PROGRAM RotaryKnifeApplication
VAR_INPUT
	RegistrationSensor				: BOOL;
END_VAR
VAR
	state							: MotionState_t;
	iTemp							: INT;
	EnableAxes						: BOOL;
	AxesEnabled						: BOOL;
	PowerWebTransport				: MC_Power;
	PowerVirtualWeb					: MC_Power;
	PowerRotaryKnife				: MC_Power;

	CoupleAxes						: BOOL;
	
	GearInVirtualWeb				: MC_GearIn;
	CamInRotaryKnife				: MC_CamIn;

	SetPositionVirtualWeb: MC_SetPosition;
	MoveModuloRotaryKnife: MC_MoveModulo;
	MoveWebTransport: MC_MoveVelocity;
	Halt: MC_Halt;

	TouchProbeRegistration: MC_TouchProbe;
	RegistrationInput : TRIGGER_REF;
	RegistrationError: LREAL;
	ExpectedRegistrationPosition: LREAL;

	MoveSuperImposedVirtualWeb: MC_MoveSuperImposed;
	VirtualWebSyncAngle: LREAL;
	TriggerRegistrationCorrection: R_TRIG;
	TriggerCorrectionFinished : R_TRIG;
	
	lrSlavepos: LREAL;
	
	fbPosTrig:Tc2_Standard.R_TRIG;
END_VAR


(* rotary knife state machine *)

CASE state OF
	MOTIONSTATE_INIT :  //Init
		EnableAxes := FALSE;
		CoupleAxes := FALSE;
		SetPositionVirtualWeb.Execute := FALSE;
		MoveModuloRotaryKnife.Execute := FALSE;
		MoveWebTransport.Execute := FALSE;
		RotaryKnifeCamTable(Execute:=FALSE);
		state := MOTIONSTATE_ADJUSTCAMTABLE ;

	MOTIONSTATE_ADJUSTCAMTABLE :   //CamData
		RotaryKnifeCamTable(Execute:=TRUE , ProductLength:=PRODUCTLENGTH );
		IF RotaryKnifeCamTable.Done THEN
			state := MOTIONSTATE_ENABLE ;
		END_IF

	MOTIONSTATE_ENABLE :        //RegulateOn
		EnableAxes := TRUE;
		IF AxesEnabled THEN
			state := MOTIONSTATE_MOVESLAVE ;
		END_IF

	MOTIONSTATE_MOVESLAVE :   //VirtualMaster to 0 ; Knife Move
		SetPositionVirtualWeb.Execute := TRUE;
		MoveModuloRotaryKnife.Execute := TRUE;
		IF SetPositionVirtualWeb.Done AND MoveModuloRotaryKnife.Done THEN
			state := MOTIONSTATE_COUPLE ;
		END_IF

	MOTIONSTATE_COUPLE :  // Couple  Master Vel With VirtualMaster ;   VirtualMaster Cam With Knife
		CoupleAxes := TRUE;
		IF CamInRotaryKnife.InSync THEN
			state := MOTIONSTATE_START ;
		END_IF

	MOTIONSTATE_START :   // Master Move
		MoveWebTransport.Execute := TRUE;

	MOTIONSTATE_ERROR :
		;
	MOTIONSTATE_RESET :
		;
END_CASE

ActPower();
ActCoupleAxes();
ActMoveSlave();
ActMoveMaster();
ActRegistration();

ACTION ActCoupleAxes:
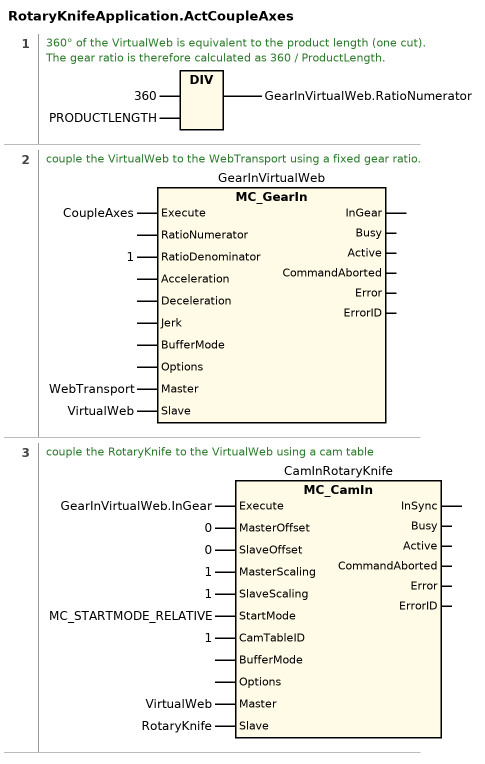
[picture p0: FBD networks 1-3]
// NETWORK 1
// 					360° of the VirtualWeb is equivalent to the product length (one cut).
// The gear ratio is therefore calculated as 360 / ProductLength.
//
GearInVirtualWeb.RatioNumerator := 360 / PRODUCTLENGTH;

// NETWORK 2
// 					couple the VirtualWeb to the WebTransport using a fixed gear ratio.
//
//
GearInVirtualWeb(Execute := CoupleAxes, RatioDenominator := 1, Master := WebTransport, Slave := VirtualWeb); // MC_GearIn

// NETWORK 3
// 					couple the RotaryKnife to the VirtualWeb using a cam table
//
//
CamInRotaryKnife(
    Execute := GearInVirtualWeb.InGear,
    MasterOffset := 0,
    SlaveOffset := 0,
    MasterScaling := 1,
    SlaveScaling := 1,
    StartMode := MC_STARTMODE_RELATIVE,
    CamTableID := 1,
    Master := VirtualWeb,
    Slave := RotaryKnife); // MC_CamIn
END_ACTION

ACTION ActMoveMaster:
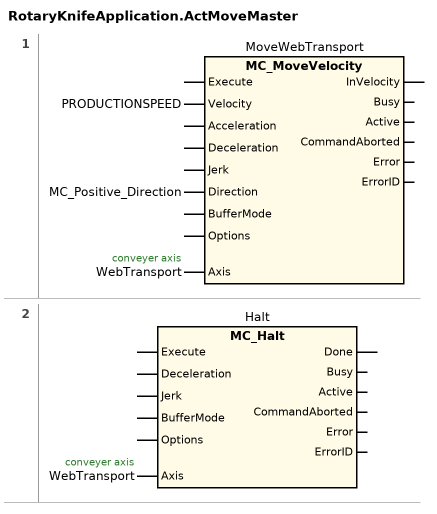
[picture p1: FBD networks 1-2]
// NETWORK 1
//   WebTransport: conveyer axis
MoveWebTransport(Velocity := PRODUCTIONSPEED, Direction := MC_Positive_Direction, Axis := WebTransport); // MC_MoveVelocity

// NETWORK 2
//   WebTransport: conveyer axis
Halt(Axis := WebTransport); // MC_Halt
END_ACTION

ACTION ActMoveSlave:
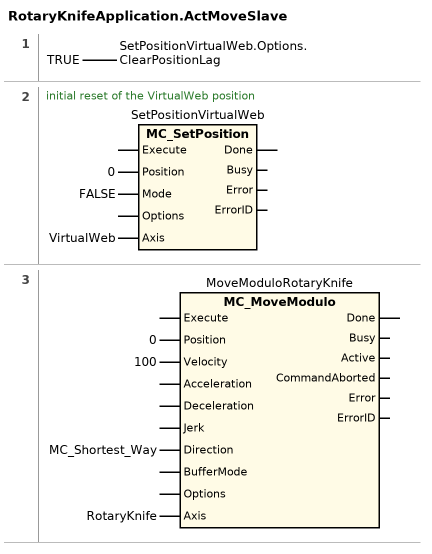
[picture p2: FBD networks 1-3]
// NETWORK 1
SetPositionVirtualWeb.Options.ClearPositionLag := TRUE;

// NETWORK 2
// 					initial reset of the VirtualWeb position
//
//
SetPositionVirtualWeb(Position := 0, Mode := FALSE, Axis := VirtualWeb); // MC_SetPosition

// NETWORK 3
MoveModuloRotaryKnife(Position := 0, Velocity := 100, Direction := MC_Shortest_Way, Axis := RotaryKnife); // MC_MoveModulo
END_ACTION

ACTION ActPower:
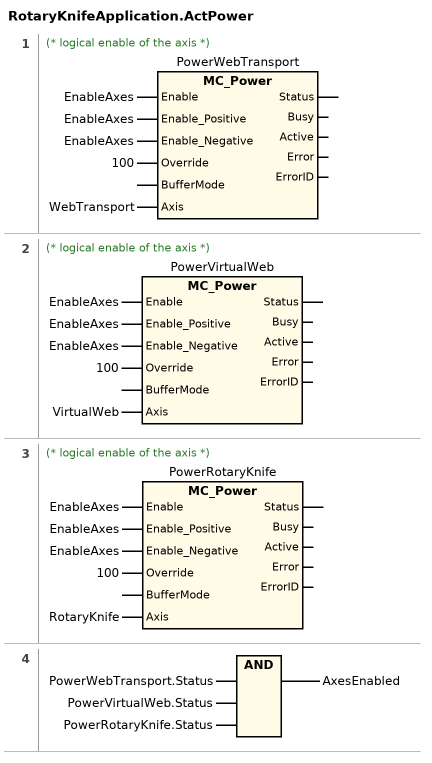
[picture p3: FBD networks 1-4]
// NETWORK 1
// (* logical enable of the axis *)
PowerWebTransport(
    Enable := EnableAxes,
    Enable_Positive := EnableAxes,
    Enable_Negative := EnableAxes,
    Override := 100,
    Axis := WebTransport); // MC_Power

// NETWORK 2
// (* logical enable of the axis *)
PowerVirtualWeb(
    Enable := EnableAxes,
    Enable_Positive := EnableAxes,
    Enable_Negative := EnableAxes,
    Override := 100,
    Axis := VirtualWeb); // MC_Power

// NETWORK 3
// (* logical enable of the axis *)
PowerRotaryKnife(
    Enable := EnableAxes,
    Enable_Positive := EnableAxes,
    Enable_Negative := EnableAxes,
    Override := 100,
    Axis := RotaryKnife); // MC_Power

// NETWORK 4
AxesEnabled := PowerWebTransport.Status AND PowerVirtualWeb.Status AND PowerRotaryKnife.Status;
END_ACTION

ACTION ActRegistration:
(*
 * 	The registration routine detects the registration sensor 
 *	and calculates a position error. The error is corrected by
 *	shifting the VirtualWeb against the WebTransport.
 *)

(* define the touch probe input signal - in this case a simulated signal is used *)
RegistrationInput.Edge := RisingEdge;
RegistrationInput.EncoderID := REGISTRATIONENCODERID;
RegistrationInput.ModuloPositions := TRUE;
RegistrationInput.TouchProbe := PlcEvent; (* use simulated PLC signal, no real probe signal *)

(* feed registration sensor *)
RegistrationInput.PlcEvent := RegistrationSensor; (* simulated PLC signal *)

(* call the registration sensor function block *)
ActRegistrationTouchProbe();

(* calculate a position error after the registration sensor triggered *)
IF 	TouchProbeRegistration.Done	(* new registration value *)
	AND NOT MoveSuperImposedVirtualWeb.Busy (* do not calculate a registration error while correction is busy (wrong measurement) *)
	THEN
	iTemp:=itemp+1;
	ExpectedRegistrationPosition := (PRODUCTLENGTH - REGISTRATIONSENSORDISTANCE) / PRODUCTLENGTH * 360.0;
	RegistrationError := ExpectedRegistrationPosition - TouchProbeRegistration.RecordedPosition;
END_IF

(* registration correction - shift the VirtualWeb against the WebTransport *)
VirtualWebSyncAngle := ROTARYKNIFESYNCANGLE / PRODUCTLENGTH * ROTARYKNIFECIRCUMFERENCE;
TriggerRegistrationCorrection( CLK:= VirtualWeb.NcToPlc.ModuloSetPos > VirtualWebSyncAngle);
IF TriggerRegistrationCorrection.Q AND ABS(RegistrationError)>0.1 THEN
	(* start correction when the rotaray knife leaves the synchronized cutting range *)
	MoveSuperImposedVirtualWeb.Length := 360 - VirtualWebSyncAngle - VirtualWeb.NcToPlc.ModuloSetPos;	(* available range for registration correction *)
	MoveSuperImposedVirtualWeb.Distance := RegistrationError; (* registration correction value *)
	MoveSuperImposedVirtualWeb.VelocityDiff := VirtualWeb.NcToPlc.SetVelo / 30; (* maximum allowed change of velocity e. g. 10% *)
	MoveSuperImposedVirtualWeb.Execute := TRUE; (* start corection *)
	RegistrationError := 0; (* reset value *)
ELSIF VirtualWeb.NcToPlc.ModuloSetPos > (360 - VirtualWebSyncAngle) THEN
	(* axis reached synchrounous range before cutting *)
	MoveSuperImposedVirtualWeb.Execute := FALSE; (* reset block *)
END_IF

(* call the registration correction function block *)
ActRegistrationCorrection();
TriggerCorrectionFinished(CLK:=MoveSuperImposedVirtualWeb.Done OR MoveSuperImposedVirtualWeb.Warning);
IF TriggerCorrectionFinished.Q THEN
	CumulatedRegistrationError := CumulatedRegistrationError + MoveSuperImposedVirtualWeb.ActualDistance;
END_IF
END_ACTION

ACTION ActRegistrationCorrection:
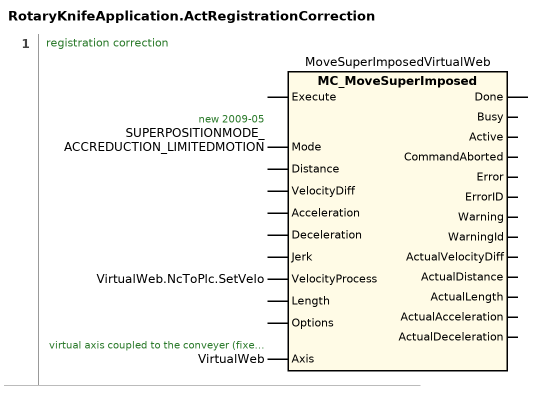
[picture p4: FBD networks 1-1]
// NETWORK 1
// registration correction
//   SUPERPOSITIONMODE_ACCREDUCTION_LIMITEDMOTION: new 2009-05
//   VirtualWeb: virtual axis coupled to the conveyer (fixed gear ratio)
MoveSuperImposedVirtualWeb(
    Mode := SUPERPOSITIONMODE_ACCREDUCTION_LIMITEDMOTION,
    VelocityProcess := VirtualWeb.NcToPlc.SetVelo,
    Axis := VirtualWeb); // MC_MoveSuperImposed
END_ACTION

ACTION ActRegistrationTouchProbe:
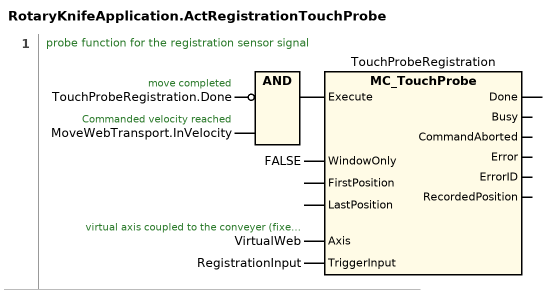
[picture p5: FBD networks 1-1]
// NETWORK 1
// 					probe function for the registration sensor signal
//
//
//   TouchProbeRegistration.Done: move completed
//   MoveWebTransport.InVelocity: Commanded velocity reached
//   VirtualWeb: virtual axis coupled to the conveyer (fixed gear ratio)
TouchProbeRegistration(
    Execute := NOT TouchProbeRegistration.Done AND MoveWebTransport.InVelocity,
    WindowOnly := FALSE,
    Axis := VirtualWeb,
    TriggerInput := RegistrationInput); // MC_TouchProbe
END_ACTION

END_PROGRAM
